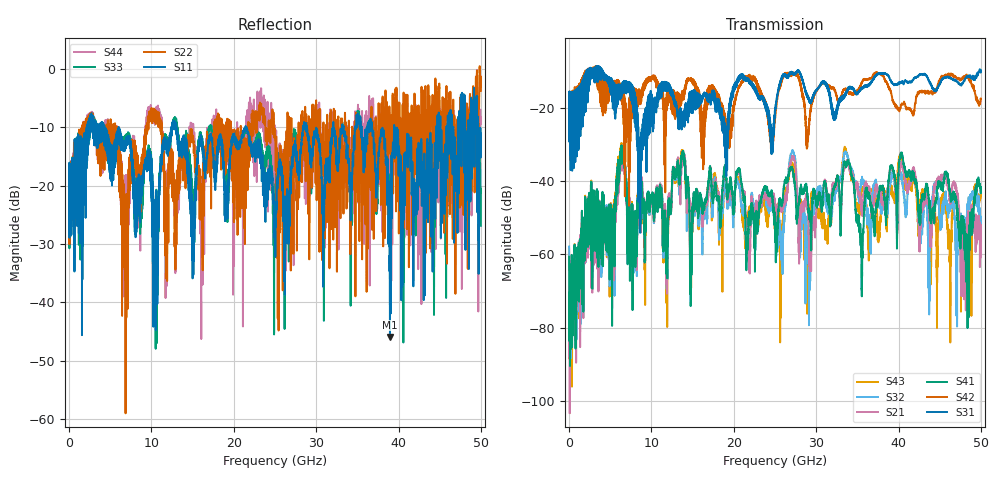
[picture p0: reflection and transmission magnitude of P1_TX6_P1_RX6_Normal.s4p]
!Keysight Technologies,N5225B,MY57041031,A.13.20.10
!Date: Friday, May 31, 2019 11:22:45
!Correction: S11(Full 4 Port(1,2,3,4))
!S12(Full 4 Port(1,2,3,4))
!S13(Full 4 Port(1,2,3,4))
!S14(Full 4 Port(1,2,3,4))
!S21(Full 4 Port(1,2,3,4))
!S22(Full 4 Port(1,2,3,4))
!S23(Full 4 Port(1,2,3,4))
!S24(Full 4 Port(1,2,3,4))
!S31(Full 4 Port(1,2,3,4))
!S32(Full 4 Port(1,2,3,4))
!S33(Full 4 Port(1,2,3,4))
!S34(Full 4 Port(1,2,3,4))
!S41(Full 4 Port(1,2,3,4))
!S42(Full 4 Port(1,2,3,4))
!S43(Full 4 Port(1,2,3,4))
!S44(Full 4 Port(1,2,3,4))
!S4P File: Measurements: <S11,S12,S13,S14>,
!<S21,S22,S23,S24>,
!<S31,S32,S33,S34>,
!<S41,S42,S43,S44>:
# Hz S  dB  R 50.0
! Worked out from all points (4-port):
!   5000 points, 10 MHz to 50 GHz, reference 50 ohm
!   strongest paths, dB at 10 MHz, 12.51 GHz, 25.01 GHz, 37.51 GHz, 50 GHz:
!     S31: -19.3, -15.5, -21.6, -10.8, -9.9
!     S42: -19.4, -15.6, -23.0, -10.7, -17.8
!     S41: -60.6, -39.7, -53.7, -44.7, -42.4
!     S21: -76.0, -40.7, -49.9, -43.2, -52.3
!     S32: -57.8, -41.1, -48.2, -45.0, -52.1
!     S43: -58.6, -40.3, -50.9, -54.1, -44.1
!   lowest |S11| = -45.9 dB at 38.96 GHz (marker M1), VSWR 1.01, Z = 50.5 + j0.133 ohm
!   |S11| at or under -10 dB: 4.286 GHz to 12.47 GHz (8.179 GHz wide, 97.6 % of centre); 13.02 GHz to 21.43 GHz (8.402 GHz wide, 48.8 % of centre); 21.46 GHz to 28.42 GHz (6.959 GHz wide, 27.9 % of centre)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
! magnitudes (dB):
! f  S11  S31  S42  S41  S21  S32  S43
! 10 MHz  -19.3  -19.3  -19.4  -60.6  -76.0  -57.8  -58.6
! 6.43 GHz  -13.1  -14.4  -18.7  -30.7  -32.1  -31.1  -30.0
! 11.68 GHz  -12.1  -13.5  -43.1  -50.5  -49.1  -51.0  -53.5
! 13.77 GHz  -12.6  -22.9  -17.2  -32.5  -33.7  -32.8  -32.0
! 21.77 GHz  -11.1  -12.2  -11.3  -54.4  -59.6  -57.1  -48.9
! 38.96 GHz  -45.9  -12.3  -14.8  -36.7  -36.8  -40.4  -41.5
! 50 GHz  -11.1  -9.9  -17.8  -42.4  -52.3  -52.1  -44.1
